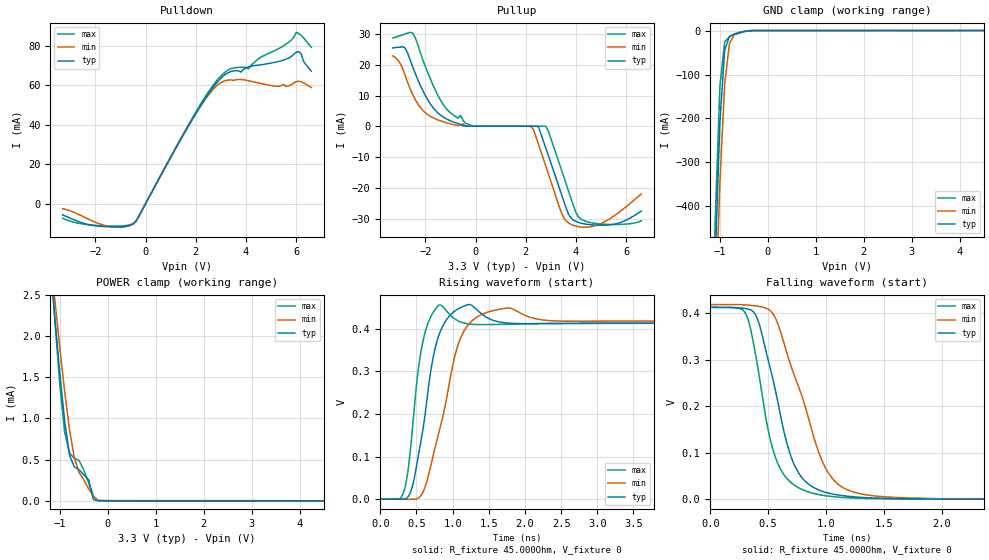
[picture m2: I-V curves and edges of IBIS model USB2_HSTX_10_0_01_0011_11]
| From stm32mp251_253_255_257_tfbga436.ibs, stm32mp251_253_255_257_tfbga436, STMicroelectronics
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[Model] USB2_HSTX_10_0_01_0011_11
Model_type   Output
Polarity   Non-Inverting
Enable   Active-High
C_comp   8.036pF   7.631pF   8.569pF
Vmeas = 200.000mV
Vref = 200.000mV
Rref = 45Ohms
Cref = 0pF
[Model Spec]
Vmeas   200.000mV   200.000mV   200.000mV
Vref   200.000mV   200.000mV   200.000mV
| This model is not intended for timing simulations.
| Warnings about Cref, Vref & Rref can be ignored
[Temperature Range]   25.000   125.000   -40.000
[Voltage Range]   3.300V   3.070V   3.630V
[GND Clamp Reference]   0.00V   0.00V   0.00V
[Pulldown Reference]   0.00V   0.00V   0.00V
[POWER Clamp Reference]   3.300V   3.070V   3.630V
[Pullup Reference]   3.300V   3.070V   3.630V
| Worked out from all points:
|   slope of the pulldown table from 0 to 0.495 V, typ, clamps not added: 42.6 ohm
|   GND clamp passes 1 mA (typ) near -0.43 V on its own axis
|   POWER clamp passes 1 mA (typ) near -0.91 V on its own axis
|   rising waveform, R_fixture 45.000Ohm, V_fixture 0: 20-80 % time 222ps typ, 324ps min, 152ps max; typ from 0 V to 0.413 V
|   falling waveform, R_fixture 45.000Ohm, V_fixture 0: 20-80 % time 242ps typ, 327ps min, 197ps max; typ from 0.413 V to 0 V
[GND Clamp]
-3.3V     -11.02A    -10.62A    -11.32A
-1.2V     -931.6mA   -1.049A    -855.7mA
-1.1V     -533.1mA   -671.7mA   -440.2mA
-1V       -209.4mA   -347mA     -127.3mA
-900mV    -44.44mA   -121.7mA   -25.6mA
-800mV    -13.15mA   -29.48mA   -14.15mA
-700mV    -7.743mA   -9.125mA   -9.769mA
-500mV    -2.127mA   -1.981mA   -2.894mA
-300mV    -19.47uA   -62.22uA   -13.66uA
6.6V      10.37uA    26.59uA    21.05uA
[Power Clamp]
-3.3V     3.206A     2.175A     4.855A
-1.2V     2.88mA     3.008mA    2.969mA
-1.1V     2.195mA    2.419mA    2.156mA
-1V       1.545mA    1.852mA    1.406mA
-900mV    967.5uA    1.324mA    831.4uA
-800mV    558.4uA    864.6uA    580.3uA
-700mV    412uA      525.9uA    517uA
-600mV    376.6uA    345uA      488.5uA
-400mV    254.2uA    146.6uA    216.8uA
-300mV    11.21uA    52.87uA    53.51uA
-100mV    94.86nA    985nA      361.1nA
6.6V      -2.721uA   -5.181uA   -3.525uA
[Pulldown]
-3.3V     -5.671mA   -2.581mA   -7.449mA
-1.6V     -11.64mA   -11.09mA   -11.31mA
-500mV    -10.25mA   -10.32mA   -10.1mA
1.9V      43.42mA    43.46mA    44.13mA
2.9V      62.15mA    60.37mA    63.26mA
3.4V      66.87mA    62.63mA    68.29mA
4.1V      69.19mA    62.19mA    68.26mA
4.5V      70.11mA    61.06mA    73.4mA
5.6V      73.12mA    59.29mA    80.76mA
6V        76.56mA    61.79mA    86.69mA
6.1V      76.96mA    61.93mA    85.99mA
6.6V      67.05mA    58.79mA    79.1mA
[Pullup]
-3.3V     25.47mA    22.87mA    28.68mA
-2.8V     25.39mA    16.38mA    30mA
-2.5V     19.21mA    10.28mA    30.28mA
-1.2V     2.603mA    1.31mA     6.11mA
-100mV    93.8uA     82.61uA    220.4uA
2.2V      68.65uA    -28.24uA   104.8uA
2.5V      -41.39uA   -5.657mA   83.46uA
2.9V      -9.472mA   -15.37mA   -1.561mA
3.5V      -23.92mA   -29.44mA   -16.02mA
3.8V      -29.68mA   -31.75mA   -23.35mA
4.4V      -31.68mA   -32.65mA   -30.79mA
6.6V      -27.44mA   -21.87mA   -30.63mA
[Ramp]
R_load=45.000Ohm
dV/dt_r   624.164mV/1.090ns  592.498mV/1.140ns  677.754mV/990.000ps
dV/dt_f   626.382mV/265.000ps  595.438mV/350.000ps  679.594mV/225.000ps
[Rising waveform]
R_fixture=45.000Ohm
V_fixture=0
0s        452.3nV    3.134uV    468.1nV
300ps     -354.4uV   -317.7uV   7.262mV
420ps     17.18mV    -365.6uV   121.4mV
580ps     153.7mV    13.3mV     362.9mV
710ps     313.4mV    87.09mV    432.3mV
820ps     389.4mV    162.5mV    456.1mV
1.14ns    452.1mV    389.3mV    414.3mV
1.69ns    414.8mV    447.2mV    410.7mV
2.51ns    412.4mV    418mV      412.7mV
9.9ns     413.1mV    419.1mV    412.8mV
[Falling waveform]
R_fixture=45.000Ohm
V_fixture=0
0s        412.6mV    418.6mV    412.3mV
310ps     409.6mV    417.6mV    396.7mV
410ps     385.7mV    414.9mV    283.8mV
540ps     258.8mV    398.9mV    107.5mV
650ps     130.9mV    323.5mV    48.25mV
720ps     77.02mV    269.7mV    31.48mV
970ps     16.9mV     80mV       8.645mV
1.18ns    6.737mV    20.81mV    3.437mV
1.68ns    1.211mV    3.228mV    832uV
9.9ns     13.72uV    31.37uV    3.564uV
